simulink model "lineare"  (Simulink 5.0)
settings: Solver=ode45  StartTime=0.0  StopTime=1000  RelTol=1e-3
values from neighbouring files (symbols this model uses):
  a = 1    [Evani.m]
  Cx = 0.8    [Evani.m]
  Fx1 = 800    [Evani.m]
  Fy1 = 400    [Evani.m]
  J = 300    [Evani.m]
  m = 540*sqrt(2)+225    [Evani.m]
  Ro = 1.5    [Evani.m]
  S = 2    [Evani.m]
  x_1 = 10    [Evani.m]
  x_2 = -1/(m*x_3)*(Fx1*cos(pi/4)+Fx2-Fy1*sin(pi/4)-Ro*S*Cx*x_1^2/2)    [Evani.m]
  x_3 = x_1/Ra    (= 0.111111111111)    [Evani.m]
undefined symbols (not defined in the file or in its folder): Ar, Br, Cr, Dr

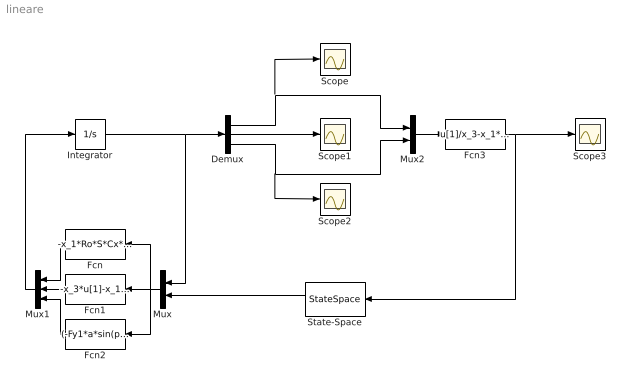
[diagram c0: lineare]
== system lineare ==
  Demux : Demux  Outputs=3
  Fcn : Fcn  Orientation=left  Expr=-x_1*Ro*S*Cx*u[1]/m+x_3*u[2]+x_2*u[3]-(Fx1*sin(pi/4)+Fy1*cos(pi/4))*u[4]/m
  Fcn1 : Fcn  Orientation=left  Expr=-x_3*u[1]-x_1*u[3]+(-Fy1*sin(pi/4)+Fx1*cos(pi/4))*u[4]/m
  Fcn2 : Fcn  Orientation=left  Expr=(-Fy1*a*sin(pi/4)+Fx1*a*cos(pi/4))*u[4]/J
  Fcn3 : Fcn  Expr=u[1]/x_3-x_1*u[2]/x_3^2
  Integrator : Integrator  InitialCondition=[0;0;1]
  Mux : Mux  Orientation=left  Inputs=2
  Mux1 : Mux  Orientation=left  Inputs=3
  Mux2 : Mux  Inputs=2
  Scope{,1..3} (4 alike) : Scope
  State-Space : StateSpace  Orientation=left  A=Ar  B=Br  C=Cr  D=Dr  X0=[0;0;0]
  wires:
  Fcn2/1 -> Mux1/3
  Fcn1/1 -> Mux1/2
  Fcn/1 -> Mux1/1
  Mux2/1 -> Fcn3/1
  Mux1/1 -> Integrator/1
  Demux/2 -> Scope1/1
  State-Space/1 -> Mux/2
  Fcn3/1 -> Scope3/1, State-Space/1
  Demux/1 -> Scope/1, Mux2/1
  Demux/3 -> Mux2/2, Scope2/1
  Integrator/1 -> Demux/1, Mux/1
  Mux/1 -> Fcn1/1, Fcn/1, Fcn2/1
